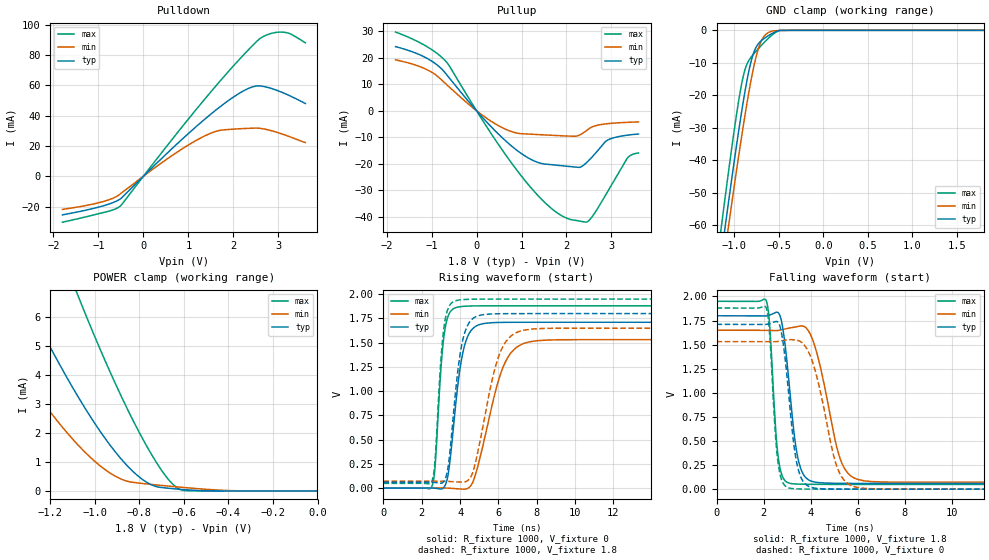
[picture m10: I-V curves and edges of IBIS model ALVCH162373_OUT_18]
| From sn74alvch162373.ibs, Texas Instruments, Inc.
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[Model]   ALVCH162373_OUT_18
Model_type  3-state
Enable   Active-Low
Vref =   0
Rref =   1000
Cref =   30p
Vmeas =   0.9
| variable   typ   min   max
C_comp   7.29pF   6.30pF   8.46pF
| C_pullup   6.47pF   4.46pF   8.84pF
| C_pulldown   5.06pF   4.16pF   5.96pF
| C_tri-state   7.29pF   6.30pF   8.46pF
[Temperature Range]   40   100   -40
| Ambient temperature   25   85   -40
[Voltage range]   1.8   1.65   1.95
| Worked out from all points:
|   slope of the pulldown table from 0 to 0.27 V, typ, clamps not added: 34.4 ohm
|   slope of the pullup table from 0 to 0.27 V, typ, clamps not added: 53.5 ohm
|   GND clamp passes 1 mA (typ) near -0.58 V on its own axis
|   POWER clamp passes 1 mA (typ) near -0.87 V on its own axis
|   rising waveform, R_fixture 1000, V_fixture 0: 20-80 % time 607ps typ, 1.17ns min, 375ps max; typ from 0 V to 1.71 V
|   falling waveform, R_fixture 1000, V_fixture 1.8: 20-80 % time 458ps typ, 818ps min, 284ps max; typ from 1.8 V to 0.059 V
|   rising waveform, R_fixture 1000, V_fixture 1.8: 20-80 % time 575ps typ, 1.03ns min, 366ps max; typ from 0.059 V to 1.8 V
|   falling waveform, R_fixture 1000, V_fixture 0: 20-80 % time 450ps typ, 825ps min, 281ps max; typ from 1.71 V to 0 V
[GND Clamp]
| ALVCH162373_OUT_18
|   Voltage   I(typ)   I(min)   I(max)
-1.8V     -210mA     -213mA     -207.3mA
-1.145V   -69.06mA   -76.1mA    -60.32mA
-1.105V   -60.89mA   -68.14mA   -51.82mA
-1.06V    -51.84mA   -59.3mA    -42.46mA
-955mV    -31.65mA   -39.36mA   -22.33mA
-880mV    -18.75mA   -26.07mA   -12.09mA
-805mV    -8.859mA   -14.32mA   -8.009mA
-740mV    -4.5mA     -6.518mA   -5.92mA
-685mV    -2.911mA   -2.612mA   -4.287mA
-620mV    -1.672mA   -727.7uA   -2.507mA
-485mV    -23.61uA   -61.14uA   -22.03uA
1.8V      60.47pA    9.421nA    28.01pA
[POWER Clamp]
| ALVCH162373_OUT_18
|   Voltage   I(typ)   I(min)   I(max)
-1.8V     15mA       10.16mA    22.87mA
-1.545V   10.46mA    6.724mA    16.81mA
-1.32V    6.769mA    4.004mA    11.77mA
-1.195V   4.893mA    2.678mA    9.129mA
-1.075V   3.254mA    1.585mA    6.738mA
-980mV    2.105mA    891.4uA    4.968mA
-900mV    1.273mA    476.4uA    3.581mA
-825mV    645.6uA    292.9uA    2.387mA
-765mV    290.1uA    239.7uA    1.523mA
-685mV    104.9uA    178.3uA    548.2uA
-620mV    56.95uA    132.3uA    61.78uA
-16.28fV  60.47pA    287pA      33.61pA
[Pulldown]
| ALVCH162373_OUT_18
|   Voltage   I(typ)   I(min)   I(max)
-1.8V     -25.46mA   -21.84mA   -30.29mA
-920mV    -19.74mA   -16.91mA   -24.15mA
-655mV    -17.11mA   -14.24mA   -21.96mA
-505mV    -14.79mA   -11.45mA   -19.4mA
555mV     15.94mA    11.96mA    21.16mA
1.295V    35.84mA    25.55mA    48.36mA
1.705V    45.8mA     30.27mA    62.74mA
2.32V     57.68mA    31.54mA    82.88mA
2.62V     59.41mA    31.45mA    91.32mA
2.955V    56.74mA    29.06mA    94.82mA
3.245V    53.15mA    26.12mA    94.08mA
3.6V      47.92mA    22.21mA    87.94mA
[Pullup]
| ALVCH162373_OUT_18
|   Voltage   I(typ)   I(min)   I(max)
-1.8V     24.15mA    19.17mA    29.63mA
-1.115V   19.87mA    15.59mA    24.29mA
-685mV    14.02mA    10.16mA    18.67mA
215mV     -4.052mA   -2.712mA   -5.747mA
875mV     -14.61mA   -8.332mA   -21.91mA
1.365V    -19.49mA   -8.984mA   -31.94mA
1.95V     -20.81mA   -9.486mA   -40.07mA
2.295V    -21.33mA   -9.107mA   -41.58mA
2.485V    -18.9mA    -6.977mA   -41.56mA
2.915V    -11.06mA   -4.876mA   -30.45mA
3.355V    -9.207mA   -4.37mA    -17.82mA
3.6V      -8.773mA   -4.223mA   -15.91mA
[Ramp]
| ALVCH162373_OUT_18
| variable   typ   min   max
dV/dt_r   1.03/6.15E-10   0.93/1.18E-09   1.13/3.80E-10
dV/dt_f   1.07/4.74E-10   0.97/8.46E-10   1.15/2.91E-10
R_load = 1000
[Rising Waveform]
| ALVCH162373_OUT_18
R_fixture =   1000
C_fixture =   0
L_fixture =   0
V_fixture =   0
V_fixture_min = 0
V_fixture_max = 0
|   Time   V(typ)   V(min)   V(max)
0s        309.1pV    1.643nV    216.2pV
2.535ns   717.8uV    719uV      21.32mV
2.695ns   -1.057mV   863.8uV    223.4mV
3.16ns    8.537mV    925.9uV    1.569V
3.735ns   791.4mV    -4.855mV   1.859V
4.12ns    1.374V     -10.1mV    1.874V
4.58ns    1.627V     31.11mV    1.879V
6.175ns   1.709V     1.214V     1.881V
7.325ns   1.711V     1.492V     1.881V
24.99ns   1.711V     1.532V     1.881V
[Falling Waveform]
| ALVCH162373_OUT_18
R_fixture =   1000
C_fixture =   0
L_fixture =   0
V_fixture =   1.8
V_fixture_min = 1.65
V_fixture_max = 1.95
|   Time   V(typ)   V(min)   V(max)
0s        1.8V       1.65V      1.95V
2.11ns    1.799V     1.648V     1.961V
2.255ns   1.807V     1.648V     1.711V
2.615ns   1.833V     1.648V     346.4mV
3.09ns    1.089V     1.672V     62.45mV
3.39ns    413.8mV    1.685V     53.49mV
3.72ns    142.4mV    1.689V     51.2mV
5.26ns    60.64mV    313.2mV    49.35mV
6.02ns    59.83mV    99.7mV     49.29mV
24.99ns   59.49mV    70.7mV     49.27mV
[Rising Waveform]
| ALVCH162373_OUT_18
R_fixture =   1000
C_fixture =   0
L_fixture =   0
V_fixture =   1.8
V_fixture_min = 1.65
V_fixture_max = 1.95
|   Time   V(typ)   V(min)   V(max)
0s        59.49mV    70.7mV     49.27mV
2.53ns    59.74mV    71.14mV    69.87mV
2.69ns    57.94mV    71.12mV    272.9mV
3.14ns    66.26mV    70.64mV    1.626V
3.715ns   893mV      65.29mV    1.929V
4.075ns   1.465V     62.99mV    1.943V
4.5ns     1.714V     96.99mV    1.948V
5.96ns    1.798V     1.328V     1.95V
7.035ns   1.8V       1.613V     1.95V
24.99ns   1.8V       1.65V      1.95V
[Falling Waveform]
| ALVCH162373_OUT_18
R_fixture =   1000
C_fixture =   0
L_fixture =   0
V_fixture =   0
V_fixture_min = 0
V_fixture_max = 0
|   Time   V(typ)   V(min)   V(max)
0s        1.711V     1.532V     1.881V
2.11ns    1.711V     1.531V     1.887V
2.25ns    1.718V     1.531V     1.637V
2.605ns   1.735V     1.533V     293.3mV
3.08ns    959mV      1.551V     12.26mV
3.365ns   332.7mV    1.548V     3.76mV
3.695ns   75.62mV    1.506V     1.65mV
5.12ns    940.9uV    232.5mV    71.27uV
5.875ns   235.7uV    24.76mV    16.68uV
24.99ns   -8.929nV   36.23nV    4.088nV
